| Texas Instruments Incorporated
| 6.4-GSPS Single-Channel or 3.2-GSPS Dual-Channel
| 12-Bit RF-Sampling Analog-to-Digital Converter (ADC)
| Marketing part#   ADC12DJ3200QML-SP
| Voltage Range   1.05V - 1.15V & 1.8V - 2.0V
| Package-type   CLGA [BGA]
| #pins/pkg drawing   196-pin ZMX
| CLGA Ceramic Package without columns (ceramic land grid array)
[IBIS Ver]   4.1
[File name]   adc12dj3200qml-sp_clga.ibs
[File Rev]   2.2
[Date]   12/15/2021
| Complete grounds-up generation of the IBIS model, therefore previous revision history deleted.
[Source]   Model built from spectre simulations at:
   Texas Instruments Incorporated.
   12500 TI Blvd
   Dallas, TX -75243
   Support: https://e2e.ti.com/support/data-converters/f/data-converters-forum
[Notes]
   Rev 2.0: 04/15/2021
   - all model data was revised
   - INPUT model now referring to VDD18
   - C_comp data was revised. Currently min and max values are sorted in numerical order
   (otherwise a warning is triggered by the syntax check).
   However, the max. C_comp value is derived for the IBIS min. case
   (high temp., low supply and weak process which leads to max. numerical C_comp value).
   Vice versa for min. C_comp.
   - prior NC models were replaced by TERMINATOR models which cover the clamping behaviour
   - RLC package data was revised
   - Vinl & Vinh in model SYNCB, DEVCLK and SYSREF refer to 1.1V supply
   Rev 2.1: 09/30/2021
   - corrected input pin list
   Rev 2.2: 12/15/2021
   - updates on PECL, LVDS models
   - update on OUTPUT model
[Disclaimer]  This model is designed as an aid for customers of Texas Instruments
 TI and its licensors and suppliers make no warranties, either expressed
 or implied, with respect to this  model, including the warranties of
 merchantability or fitness for a particular purpose.
 The model is provided solely on an "as is" basis. The entire risk as to
 its quality and performance is with the customer.
[Copyright] (C)Copyright 2021 Texas Instruments Incorporated.
   All rights reserved.
[Component]   ADC12DJ3200QML-SP_CLGA_PECL
[Manufacturer]  Texas Instruments Incorporated
[Package]   |196-pin ceramic BGA package
|   typ   min   max
R_pkg   1.49461   0.76102   2.43987
L_pkg   5.35n   4.13n   7.81n
C_pkg   2.29p   1.00p   3.23p
[Pin] signal_name  model_name   R_pin   L_pin   C_pin
A1   AGND   GND
A2   BG   BGCLAMP   1.32232   5.118E-09  2.691E-12
A3   AGND   GND
A4   INA+   ADCINCLAMP   1.56946   5.829E-09  1.876E-12
A5   INA-   ADCINCLAMP   1.56934   5.888E-09  1.868E-12
A6   AGND   GND
A7   NCOA0   INPUT   1.11959   4.532E-09  2.304E-12
A8   ORA0   OUTPUT   1.10657   4.934E-09  2.239E-12
A9   CALTRIG   INPUT   0.99184   4.864E-09  1.831E-12
A10   DA3+   DXCLAMP   1.47441   5.350E-09  1.954E-12
A11   DA3-   DXCLAMP   1.40462   5.275E-09  2.021E-12
A12   DA2+   DXCLAMP   1.86144   6.139E-09  2.485E-12
A13   DA2-   DXCLAMP   1.78944   6.108E-09  2.542E-12
A14   DGND   GND
B1   AGND   GND
B2   SYNCSE\   INPUT   1.76801   5.741E-09  2.797E-12
B3   AGND   GND
B4   AGND   GND
B5   AGND   GND
B6   AGND   GND
B7   NCOA1   INPUT   0.9754   4.172E-09  2.152E-12
B8   ORA1   OUTPUT   0.95631   4.449E-09  2.051E-12
B9   CALSTAT   OUTPUT   0.76102   4.700E-09  9.998E-13
B10   DA7+   DXCLAMP   1.13281   4.312E-09  1.928E-12
B11   DA7-   DXCLAMP   1.11034   4.368E-09  1.954E-12
B12   DA6+   DXCLAMP   1.58519   5.407E-09  2.154E-12
B13   DA6-   DXCLAMP   1.56666   5.246E-09  2.287E-12
B14   DGND   GND
C1   TMSTP+   SYNCB_PECL   2.43987   7.812E-09  3.212E-12
C2   VA19   POWER
C3   VA19   POWER
C4   VA19   POWER
C5   VA19   POWER
C6   AGND   GND
C7   AGND   GND
C8   DGND   GND
C9   DGND   GND
C10   VD11   POWER
C11   VD11   POWER
C12   VD11   POWER
C13   DA5+   DXCLAMP   1.38271   4.795E-09  2.158E-12
C14   DA1+   DXCLAMP   1.79966   6.012E-09  2.334E-12
D1   TMSTP-   SYNCB_PECL   2.43617   7.758E-09  3.230E-12
D2   VA19   POWER
D3   VA11   POWER
D4   AGND   GND
D5   AGND   GND
D6   AGND   GND
D7   AGND   GND
D8   DGND   GND
D9   DGND   GND
D10   DGND   GND
D11   DGND   GND
D12   VD11   POWER
D13   DA5-   DXCLAMP   1.36228   4.873E-09  2.086E-12
D14   DA1-   DXCLAMP   1.72899   5.973E-09  2.284E-12
E1   VA19   POWER
E2   VA19   POWER
E3   VA11   POWER
E4   AGND   GND
E5   AGND   GND
E6   AGND   GND
E7   AGND   GND
E8   DGND   GND
E9   DGND   GND
E10   DGND   GND
E11   DGND   GND
E12   VD11   POWER
E13   DA4+   DXCLAMP   1.09829   4.247E-09  1.849E-12
E14   DA0+   DXCLAMP   1.40206   5.007E-09  1.813E-12
F1   AGND   GND
F2   VA11   POWER
F3   VA11   POWER
F4   AGND   GND
F5   AGND   GND
F6   AGND   GND
F7   AGND   GND
F8   DGND   GND
F9   DGND   GND
F10   DGND   GND
F11   DGND   GND
F12   VD11   POWER
F13   DA4-   DXCLAMP   1.09829   4.137E-09  1.988E-12
F14   DA0-   DXCLAMP   1.26883   4.826E-09  2.006E-12
G1   CLK+   DEVCLK_PECL   1.79033   5.983E-09  2.566E-12
G2   AGND   GND
G3   VA11   POWER
G4   AGND   GND
G5   AGND   GND
G6   AGND   GND
G7   AGND   GND
G8   DGND   GND
G9   DGND   GND
G10   DGND   GND
G11   DGND   GND
G12   VD11   POWER
G13   SCS\   INPUT   1.76943   5.055E-09  2.790E-12
G14   SCLK   INPUT   1.81255   5.220E-09  2.850E-12
H1   CLK-   DEVCLK_PECL   1.79043   5.977E-09  2.578E-12
H2   AGND   GND
H3   VA11   POWER
H4   AGND   GND
H5   AGND   GND
H6   AGND   GND
H7   AGND   GND
H8   DGND   GND
H9   DGND   GND
H10   DGND   GND
H11   DGND   GND
H12   VD11   POWER
H13   SDI   INPUT   1.7713   5.080E-09  2.788E-12
H14   SDO   OUTPUT   1.89915   5.373E-09  2.949E-12
J1   AGND   GND
J2   VA11   POWER
J3   VA11   POWER
J4   AGND   GND
J5   AGND   GND
J6   AGND   GND
J7   AGND   GND
J8   DGND   GND
J9   DGND   GND
J10   DGND   GND
J11   DGND   GND
J12   VD11   POWER
J13   DB4-   DXCLAMP   1.08092   4.133E-09  1.991E-12
J14   DB0-   DXCLAMP   1.26954   4.813E-09  1.995E-12
K1   VA19   POWER
K2   VA19   POWER
K3   VA11   POWER
K4   AGND   GND
K5   AGND   GND
K6   AGND   GND
K7   AGND   GND
K8   DGND   GND
K9   DGND   GND
K10   DGND   GND
K11   DGND   GND
K12   VD11   POWER
K13   DB4+   DXCLAMP   1.0992   4.240E-09  1.876E-12
K14   DB0+   DXCLAMP   1.40228   5.005E-09  1.809E-12
L1   SYSREF+   SYSREF_PECL   2.41893   7.557E-09  3.231E-12
L2   VA19   POWER
L3   VA11   POWER
L4   AGND   GND
L5   AGND   GND
L6   AGND   GND
L7   AGND   GND
L8   DGND   GND
L9   DGND   GND
L10   DGND   GND
L11   DGND   GND
L12   VD11   POWER
L13   DB5-   DXCLAMP   1.35893   4.878E-09  2.106E-12
L14   DB1-   DXCLAMP   1.72882   5.945E-09  2.297E-12
M1   SYSREF-   SYSREF_PECL   2.42225   7.435E-09  3.232E-12
M2   VA19   POWER
M3   VA19   POWER
M4   VA19   POWER
M5   VA19   POWER
M6   AGND   GND
M7   AGND   GND
M8   DGND   GND
M9   DGND   GND
M10   VD11   POWER
M11   VD11   POWER
M12   VD11   POWER
M13   DB5+   DXCLAMP   1.3846   4.791E-09  2.194E-12
M14   DB1+   DXCLAMP   1.79944   6.001E-09  2.355E-12
N1   AGND   GND
N2   TDIODE+   TDCLAMP   2.02809   6.248E-09  3.203E-12
N3   AGND   GND
N4   AGND   GND
N5   AGND   GND
N6   AGND   GND
N7   NCOB1   INPUT   1.00982   4.258E-09  2.320E-12
N8   ORB1   OUTPUT   0.88878   4.131E-09  2.133E-12
N9   DGND   GND
N10   DB7+   DXCLAMP   1.13367   4.315E-09  1.922E-12
N11   DB7-   DXCLAMP   1.11047   4.367E-09  1.955E-12
N12   DB6+   DXCLAMP   1.58643   5.398E-09  2.149E-12
N13   DB6-   DXCLAMP   1.57026   5.254E-09  2.271E-12
N14   DGND   GND
P1   AGND   GND
P2   TDIODE-   TDCLAMP   2.02749   6.279E-09  3.204E-12
P3   AGND   GND
P4   INB+   ADCINCLAMP   1.56962   5.767E-09  1.886E-12
P5   INB-   ADCINCLAMP   1.56966   5.764E-09  1.895E-12
P6   AGND   GND
P7   NCOB0   INPUT   1.10539   4.748E-09  2.420E-12
P8   ORB0   OUTPUT   1.00643   4.728E-09  2.261E-12
P9   PD   INPUT   0.94503   5.595E-09  1.587E-12
P10   DB3+   DXCLAMP   1.47622   5.347E-09  1.927E-12
P11   DB3-   DXCLAMP   1.40395   5.250E-09  2.023E-12
P12   DB2+   DXCLAMP   1.86111   6.135E-09  2.473E-12
P13   DB2-   DXCLAMP   1.78956   6.098E-09  2.540E-12
P14   DGND   GND
[Diff pin]  inv_pin  vdiff  tdelay_typ  tdelay_min  tdelay_max
A4   A5   0.0   0.0s   0.0s   0.0s   | INA
A10   A11   0.0   0.0s   0.0s   0.0s   | DA3
A12   A13   0.0   0.0s   0.0s   0.0s   | DA2
B10   B11   0.0   0.0s   0.0s   0.0s   | DA7
B12   B13   0.0   0.0s   0.0s   0.0s   | DA6
C1   D1   0.0   0.0s   0.0s   0.0s   | TMSTP
C13   D13   0.0   0.0s   0.0s   0.0s   | DA5
C14   D14   0.0   0.0s   0.0s   0.0s   | DA1
E13   F13   0.0   0.0s   0.0s   0.0s   | DA4
E14   F14   0.0   0.0s   0.0s   0.0s   | DA0
G1   H1   0.0   0.0s   0.0s   0.0s   | DEVCLK
K13   J13   0.0   0.0s   0.0s   0.0s   | DB4
K14   J14   0.0   0.0s   0.0s   0.0s   | DB0
L1   M1   0.0   0.0s   0.0s   0.0s   | SYSREF
M13   L13   0.0   0.0s   0.0s   0.0s   | DB5
M14   L14   0.0   0.0s   0.0s   0.0s   | DB1
N10   N11   0.0   0.0s   0.0s   0.0s   | DB7
N12   N13   0.0   0.0s   0.0s   0.0s   | DB6
P4   P5   0.0   0.0s   0.0s   0.0s   | INB
P10   P11   0.0   0.0s   0.0s   0.0s   | DB3
P12   P13   0.0   0.0s   0.0s   0.0s   | DB2
[Component]   ADC12DJ3200QML-SP_CLGA_LVDS
[Manufacturer]  Texas Instruments Incorporated
[Package]   |196-pin ceramic BGA package
|   typ   min   max
R_pkg   1.49461   0.76102   2.43987
L_pkg   5.35n   4.13n   7.81n
C_pkg   2.29p   1.00p   3.23p
[Pin] signal_name  model_name   R_pin   L_pin   C_pin
A1   AGND   GND
A2   BG   BGCLAMP   1.32232   5.118E-09  2.691E-12
A3   AGND   GND
A4   INA+   ADCINCLAMP   1.56946   5.829E-09  1.876E-12
A5   INA-   ADCINCLAMP   1.56934   5.888E-09  1.868E-12
A6   AGND   GND
A7   NCOA0   INPUT   1.11959   4.532E-09  2.304E-12
A8   ORA0   OUTPUT   1.10657   4.934E-09  2.239E-12
A9   CALTRIG   INPUT   0.99184   4.864E-09  1.831E-12
A10   DA3+   DXCLAMP   1.47441   5.350E-09  1.954E-12
A11   DA3-   DXCLAMP   1.40462   5.275E-09  2.021E-12
A12   DA2+   DXCLAMP   1.86144   6.139E-09  2.485E-12
A13   DA2-   DXCLAMP   1.78944   6.108E-09  2.542E-12
A14   DGND   GND
B1   AGND   GND
B2   SYNCSE\   INPUT   1.76801   5.741E-09  2.797E-12
B3   AGND   GND
B4   AGND   GND
B5   AGND   GND
B6   AGND   GND
B7   NCOA1   INPUT   0.9754   4.172E-09  2.152E-12
B8   ORA1   OUTPUT   0.95631   4.449E-09  2.051E-12
B9   CALSTAT   OUTPUT   0.76102   4.700E-09  9.998E-13
B10   DA7+   DXCLAMP   1.13281   4.312E-09  1.928E-12
B11   DA7-   DXCLAMP   1.11034   4.368E-09  1.954E-12
B12   DA6+   DXCLAMP   1.58519   5.407E-09  2.154E-12
B13   DA6-   DXCLAMP   1.56666   5.246E-09  2.287E-12
B14   DGND   GND
C1   TMSTP+   SYNCB_LVDS   2.43987   7.812E-09  3.212E-12
C2   VA19   POWER
C3   VA19   POWER
C4   VA19   POWER
C5   VA19   POWER
C6   AGND   GND
C7   AGND   GND
C8   DGND   GND
C9   DGND   GND
C10   VD11   POWER
C11   VD11   POWER
C12   VD11   POWER
C13   DA5+   DXCLAMP   1.38271   4.795E-09  2.158E-12
C14   DA1+   DXCLAMP   1.79966   6.012E-09  2.334E-12
D1   TMSTP-   SYNCB_LVDS   2.43617   7.758E-09  3.230E-12
D2   VA19   POWER
D3   VA11   POWER
D4   AGND   GND
D5   AGND   GND
D6   AGND   GND
D7   AGND   GND
D8   DGND   GND
D9   DGND   GND
D10   DGND   GND
D11   DGND   GND
D12   VD11   POWER
D13   DA5-   DXCLAMP   1.36228   4.873E-09  2.086E-12
D14   DA1-   DXCLAMP   1.72899   5.973E-09  2.284E-12
E1   VA19   POWER
E2   VA19   POWER
E3   VA11   POWER
E4   AGND   GND
E5   AGND   GND
E6   AGND   GND
E7   AGND   GND
E8   DGND   GND
E9   DGND   GND
E10   DGND   GND
E11   DGND   GND
E12   VD11   POWER
E13   DA4+   DXCLAMP   1.09829   4.247E-09  1.849E-12
E14   DA0+   DXCLAMP   1.40206   5.007E-09  1.813E-12
F1   AGND   GND
F2   VA11   POWER
F3   VA11   POWER
F4   AGND   GND
F5   AGND   GND
F6   AGND   GND
F7   AGND   GND
F8   DGND   GND
F9   DGND   GND
F10   DGND   GND
F11   DGND   GND
F12   VD11   POWER
F13   DA4-   DXCLAMP   1.09829   4.137E-09  1.988E-12
F14   DA0-   DXCLAMP   1.26883   4.826E-09  2.006E-12
G1   CLK+   DEVCLK_LVDS   1.79033   5.983E-09  2.566E-12
G2   AGND   GND
G3   VA11   POWER
G4   AGND   GND
G5   AGND   GND
G6   AGND   GND
G7   AGND   GND
G8   DGND   GND
G9   DGND   GND
G10   DGND   GND
G11   DGND   GND
G12   VD11   POWER
G13   SCS\   INPUT   1.76943   5.055E-09  2.790E-12
G14   SCLK   INPUT   1.81255   5.220E-09  2.850E-12
H1   CLK-   DEVCLK_LVDS   1.79043   5.977E-09  2.578E-12
H2   AGND   GND
H3   VA11   POWER
H4   AGND   GND
H5   AGND   GND
H6   AGND   GND
H7   AGND   GND
H8   DGND   GND
H9   DGND   GND
H10   DGND   GND
H11   DGND   GND
H12   VD11   POWER
H13   SDI   INPUT   1.7713   5.080E-09  2.788E-12
H14   SDO   OUTPUT   1.89915   5.373E-09  2.949E-12
J1   AGND   GND
J2   VA11   POWER
J3   VA11   POWER
J4   AGND   GND
J5   AGND   GND
J6   AGND   GND
J7   AGND   GND
J8   DGND   GND
J9   DGND   GND
J10   DGND   GND
J11   DGND   GND
J12   VD11   POWER
J13   DB4-   DXCLAMP   1.08092   4.133E-09  1.991E-12
J14   DB0-   DXCLAMP   1.26954   4.813E-09  1.995E-12
K1   VA19   POWER
K2   VA19   POWER
K3   VA11   POWER
K4   AGND   GND
K5   AGND   GND
K6   AGND   GND
K7   AGND   GND
K8   DGND   GND
K9   DGND   GND
K10   DGND   GND
K11   DGND   GND
K12   VD11   POWER
K13   DB4+   DXCLAMP   1.0992   4.240E-09  1.876E-12
K14   DB0+   DXCLAMP   1.40228   5.005E-09  1.809E-12
L1   SYSREF+   SYSREF_LVDS   2.41893   7.557E-09  3.231E-12
L2   VA19   POWER
L3   VA11   POWER
L4   AGND   GND
L5   AGND   GND
L6   AGND   GND
L7   AGND   GND
L8   DGND   GND
L9   DGND   GND
L10   DGND   GND
L11   DGND   GND
L12   VD11   POWER
L13   DB5-   DXCLAMP   1.35893   4.878E-09  2.106E-12
L14   DB1-   DXCLAMP   1.72882   5.945E-09  2.297E-12
M1   SYSREF-   SYSREF_LVDS   2.42225   7.435E-09  3.232E-12
M2   VA19   POWER
M3   VA19   POWER
M4   VA19   POWER
M5   VA19   POWER
M6   AGND   GND
M7   AGND   GND
M8   DGND   GND
M9   DGND   GND
M10   VD11   POWER
M11   VD11   POWER
M12   VD11   POWER
M13   DB5+   DXCLAMP   1.3846   4.791E-09  2.194E-12
M14   DB1+   DXCLAMP   1.79944   6.001E-09  2.355E-12
N1   AGND   GND
N2   TDIODE+   TDCLAMP   2.02809   6.248E-09  3.203E-12
N3   AGND   GND
N4   AGND   GND
N5   AGND   GND
N6   AGND   GND
N7   NCOB1   INPUT   1.00982   4.258E-09  2.320E-12
N8   ORB1   OUTPUT   0.88878   4.131E-09  2.133E-12
N9   DGND   GND
N10   DB7+   DXCLAMP   1.13367   4.315E-09  1.922E-12
N11   DB7-   DXCLAMP   1.11047   4.367E-09  1.955E-12
N12   DB6+   DXCLAMP   1.58643   5.398E-09  2.149E-12
N13   DB6-   DXCLAMP   1.57026   5.254E-09  2.271E-12
N14   DGND   GND
P1   AGND   GND
P2   TDIODE-   TDCLAMP   2.02749   6.279E-09  3.204E-12
P3   AGND   GND
P4   INB+   ADCINCLAMP   1.56962   5.767E-09  1.886E-12
P5   INB-   ADCINCLAMP   1.56966   5.764E-09  1.895E-12
P6   AGND   GND
P7   NCOB0   INPUT   1.10539   4.748E-09  2.420E-12
P8   ORB0   OUTPUT   1.00643   4.728E-09  2.261E-12
P9   PD   INPUT   0.94503   5.595E-09  1.587E-12
P10   DB3+   DXCLAMP   1.47622   5.347E-09  1.927E-12
P11   DB3-   DXCLAMP   1.40395   5.250E-09  2.023E-12
P12   DB2+   DXCLAMP   1.86111   6.135E-09  2.473E-12
P13   DB2-   DXCLAMP   1.78956   6.098E-09  2.540E-12
P14   DGND   GND
[Diff pin]  inv_pin  vdiff  tdelay_typ  tdelay_min  tdelay_max
A4   A5   0.0   0.0s   0.0s   0.0s   | INA
A10   A11   0.0   0.0s   0.0s   0.0s   | DA3
A12   A13   0.0   0.0s   0.0s   0.0s   | DA2
B10   B11   0.0   0.0s   0.0s   0.0s   | DA7
B12   B13   0.0   0.0s   0.0s   0.0s   | DA6
C1   D1   0.0   0.0s   0.0s   0.0s   | TMSTP
C13   D13   0.0   0.0s   0.0s   0.0s   | DA5
C14   D14   0.0   0.0s   0.0s   0.0s   | DA1
E13   F13   0.0   0.0s   0.0s   0.0s   | DA4
E14   F14   0.0   0.0s   0.0s   0.0s   | DA0
G1   H1   0.0   0.0s   0.0s   0.0s   | DEVCLK
K13   J13   0.0   0.0s   0.0s   0.0s   | DB4
K14   J14   0.0   0.0s   0.0s   0.0s   | DB0
L1   M1   0.0   0.0s   0.0s   0.0s   | SYSREF
M13   L13   0.0   0.0s   0.0s   0.0s   | DB5
M14   L14   0.0   0.0s   0.0s   0.0s   | DB1
N10   N11   0.0   0.0s   0.0s   0.0s   | DB7
N12   N13   0.0   0.0s   0.0s   0.0s   | DB6
P4   P5   0.0   0.0s   0.0s   0.0s   | INB
P10   P11   0.0   0.0s   0.0s   0.0s   | DB3
P12   P13   0.0   0.0s   0.0s   0.0s   | DB2
[Series Pin Mapping]   pin_2   model_name   function_table_group
C1   D1   100_Ohm   | SYNCB/TMSTP with 100 Ohm termination
G1   H1   100_Ohm   | DEVCLK with 100 Ohm termination
L1   M1   100_Ohm   | SYSREF with 100 Ohm termination
[Model] 100_Ohm
Model_type Series
Polarity Non-Inverting
Enable Active-High
|   typ   min   max
C_comp   0   0   0
[Voltage Range]   1.10V   1.05V   1.15V
[Temperature Range]  25   125   -40
[R Series]   100   80   120
| Models and submodels in the file (13): SYNCB_LVDS (Input), SYNCB_PECL (Input), DEVCLK_LVDS (Input), DEVCLK_PECL (Input), SYSREF_LVDS (Input), SYSREF_PECL (Input), INPUT (Input), OUTPUT (3-state), DXCLAMP (Terminator), BGCLAMP (Terminator), TDCLAMP (Terminator), ADCINCLAMP (Terminator), 100_Ohm (Series)
